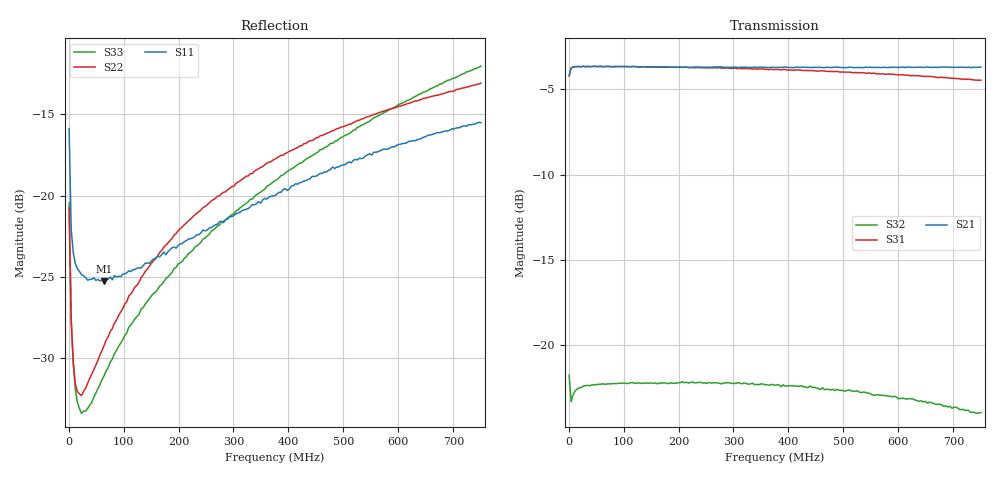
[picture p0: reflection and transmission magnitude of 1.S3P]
!Agilent Technologies,E5071B,MY42401914,A.09.10
!Date: Thu Jan 25 14:51:39 2024
!Data & Calibration Information:
!Freq	S11:SOLT3(ON)	S12:SOLT3(ON)	S13:SOLT3(ON)
!	S21:SOLT3(ON)	S22:SOLT3(ON)	S23:SOLT3(ON)
!	S31:SOLT3(ON)	S32:SOLT3(ON)	S33:SOLT3(ON)
# Hz S RI R 50
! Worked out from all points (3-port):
!   201 points, 1 MHz to 750 MHz, reference 50 ohm
!   strongest paths, dB at 1 MHz, 188.2 MHz, 375.5 MHz, 562.8 MHz, 750 MHz:
!     S21: -4.2, -3.7, -3.7, -3.7, -3.7
!     S31: -4.2, -3.7, -3.8, -4.1, -4.5
!     S32: -21.8, -22.2, -22.4, -22.9, -24.0
!   lowest |S11| = -25.3 dB at 64.67 MHz (marker M1), VSWR 1.12, Z = 45.5 + j2.68 ohm
!   |S11| at or under -10 dB: start of sweep to end of sweep
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1000000  -0.121 0.106  -0.6136 -0.0714  0.6115 0.0748
         -0.6141 -0.0717  -0.0639 0.0655  0.0726 -0.0375
         0.6121 0.0717  0.0724 -0.0375  -0.0677 0.0667
4745000  -0.0679 0.0402  -0.6498 -0.0203  0.6507 0.021
         -0.6498 -0.019  -0.0181 0.0369  0.0682 -0.0013
         0.6497 0.0208  0.0681 -0.00127  -0.0194 0.0376
8490000  -0.0603 0.0289  -0.6531 -0.00707  0.6548 0.00834
         -0.6545 -0.00611  -0.00779 0.0298  0.0717 0.00202
         0.6552 0.00706  0.0715 0.00195  -0.00858 0.0296
1.598e7  -0.0556 0.0217  -0.6559 0.00733  0.6553 -0.00515
         -0.6562 0.0077  -0.000232 0.025  0.0743 0.00199
         0.6571 -0.00605  0.0742 0.00169  -0.000626 0.0231
3.096e7  -0.0516 0.0219  -0.656 0.0268  0.6559 -0.0249
         -0.6542 0.0275  0.00538 0.025  0.0756 0.000603
         0.6558 -0.0252  0.0758 0.000544  0.00516 0.0211
6.4665e7  -0.046 0.0293  -0.6529 0.0645  0.6541 -0.059
          -0.6527 0.0616  0.0118 0.0326  0.0764 -0.00087
          0.6536 -0.0584  0.0766 -0.000844  0.0133 0.0246
1.09605e8  -0.0411 0.042  -0.6451 0.111  0.6481 -0.1021
           -0.6464 0.1094  0.0178 0.0458  0.0772 -0.0038
           0.6482 -0.1034  0.077 -0.00379  0.0221 0.0327
1.91995e8  -0.0291 0.0631  -0.6261 0.1886  0.6286 -0.1789
           -0.6255 0.1881  0.0316 0.0688  0.0768 -0.00736
           0.628 -0.1789  0.0767 -0.00763  0.0422 0.0423
3.755e8  0.00434 0.1001  -0.5501 0.3524  0.5485 -0.3331
         -0.5487 0.3528  0.0716 0.1081  0.0741 -0.0162
         0.5498 -0.3348  0.0744 -0.016  0.1055 0.0353
7.5e8  0.0962 0.1375  -0.2835 0.5888  0.2651 -0.5369
       -0.2833 0.5899  0.1776 0.1332  0.0567 -0.0274
       0.2657 -0.5364  0.057 -0.0275  0.2148 -0.1285
